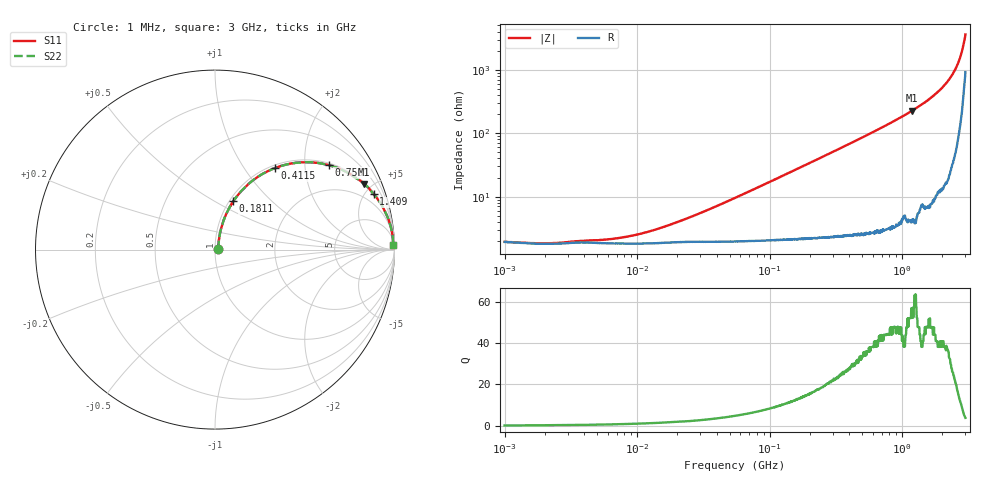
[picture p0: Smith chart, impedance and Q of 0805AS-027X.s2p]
!s-Parameter Generated by FASTRON Sdn. Bhd.
!FASTRON P/N : 0805AS-027X
!Keysight Technologies: E4991B_MY54100416_A.01.15
!Date: Mon Jun 15 12:49:49 2026
!Version  :Rev01  Mon Jun 15 12:49:49 2026
!Data & Calibration Information:
!Freq  S11  S21  S12  S22
!PortZ  Port1:50+j0  Port2:50+j0
!When reading reference impedance value at option line is always used.
! Remarks : This data is being provided solely for informational purposes.
# Hz S dB R 50
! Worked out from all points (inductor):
!   1601 points, 1 MHz to 3 GHz, reference 50 ohm
!   read as one part in series: L = 27.3 nH near 33.88 MHz
!   highest Q = 52.4 at 1.189 GHz (marker M1), where L = 30.3 nH
!   S11 on the Smith chart (normalised r, x): 1 MHz: 1.04, +0.00; 181.1 MHz: 1.04, +0.61; 411.5 MHz: 1.05, +1.40; 750.1 MHz: 1.06, +2.64; 1.409 GHz: 1.14, +5.69; 3 GHz: 19, +70
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1000000  -34.40 5.2  -0.17 -0.1  -0.17 -0.1  -34.40 5.2
2014875  -34.90 11.0  -0.15 -0.2  -0.15 -0.2  -34.90 11.0
3804036  -34.10 19.2  -0.16 -0.4  -0.16 -0.4  -34.10 19.2
7327130  -33.20 34.5  -0.16 -0.7  -0.16 -0.7  -33.20 34.5
1.447069e7  -30.30 52.3  -0.16 -1.4  -0.16 -1.4  -30.30 52.3
2.572808e7  -26.50 63.9  -0.17 -2.5  -0.17 -2.5  -26.50 63.9
5.504702e7  -20.60 72.9  -0.21 -5.3  -0.21 -5.3  -20.60 72.9
1.034087e8  -15.40 73.6  -0.30 -9.8  -0.30 -9.8  -15.40 73.6
1.811155e8  -10.80 69.3  -0.56 -16.7  -0.56 -16.7  -10.80 69.3
2.083556e8  -9.72 67.4  -0.68 -19.0  -0.68 -19.0  -9.72 67.4
2.92808e8  -7.20 61.5  -1.11 -25.8  -1.11 -25.8  -7.20 61.5
4.114912e8  -4.96 53.6  -1.88 -34.4  -1.88 -34.4  -4.96 53.6
5.611759e8  -3.28 45.2  -2.98 -43.3  -2.98 -43.3  -3.28 45.2
7.50144e8  -2.06 36.7  -4.48 -52.0  -4.48 -52.0  -2.06 36.7
7.925923e8  -1.87 35.0  -4.82 -53.7  -4.82 -53.7  -1.87 35.0
1.188719e9  -0.83 23.7  -7.93 -65.3  -7.93 -65.3  -0.83 23.7
1.409185e9  -0.57 19.2  -9.68 -69.3  -9.68 -69.3  -0.57 19.2
1.902655e9  -0.24 12.0  -13.70 -76.5  -13.70 -76.5  -0.24 12.0
2.324278e9  -0.11 7.4  -17.80 -80.7  -17.80 -80.7  -0.11 7.4
2.660507e9  -0.07 4.3  -22.50 -81.8  -22.50 -81.8  -0.07 4.3
2.783064e9  -0.06 3.3  -24.90 -81.3  -24.90 -81.3  -0.06 3.3
3e9  -0.06 1.5  -31.20 -73.7  -31.20 -73.7  -0.06 1.5
